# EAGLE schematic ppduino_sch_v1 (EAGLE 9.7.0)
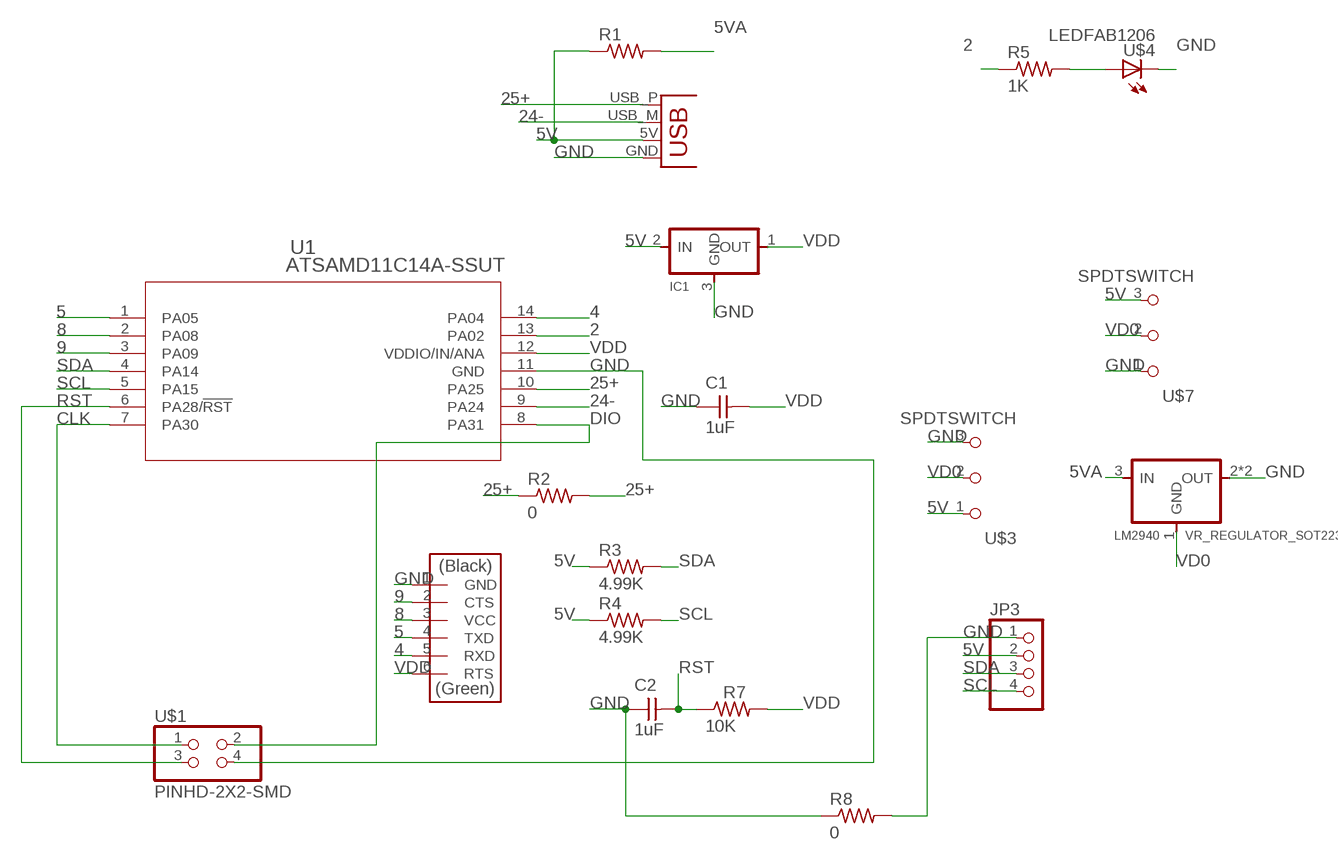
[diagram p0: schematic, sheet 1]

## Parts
C1  1uF  CAP_UNPOLARIZEDFAB  [C1206FAB]
C2  1uF  CAP_UNPOLARIZEDFAB  [C1206FAB]
IC1  VR_REGULATOR-SOT23SOT23  [SOT23]
JP3  PINHD-1X04_2.54-SMD-90°  [1X04SMD/90]
LM2940  VR_REGULATOR_SOT223  [SOT223]
R1  RES-US1206FAB  [R1206FAB]
R2  0  R1206FAB  [R1206FAB]
R3  4.99K  R1206FAB  [R1206FAB]
R4  4.99K  R1206FAB  [R1206FAB]
R5  1K  R1206FAB  [R1206FAB]
R7  10K  R1206FAB  [R1206FAB]
R8  0  R1206FAB  [R1206FAB]
U1  ATSAMD11C14A-SSUT  [SOIC14_SL_MCH]
U$1  PINHD-2X2-SMD  [2X02SMD]
U$3  SPDTSWITCH  [SPDTSWITCH]
U$4  LEDFAB1206  [LED1206FAB]
U$6  CONN_06_FTDI-SMD-HEADER  [1X06SMD]
U$7  SPDTSWITCH  [SPDTSWITCH]
X1  CONN_USBPCB  [USB-A-PCB]

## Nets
2: R5.1 U1.13(PA02)
4: U1.14(PA04) U$6.5(RXD)
5: U1.1(PA05) U$6.4(TXD)
5V: IC1.2(IN) JP3.2 R1.1 R3.1 R4.1 U$3.1 U$7.3 X1.5V(VBUS)
5VA: LM2940.3(IN) R1.2
8: U1.2(PA08) U$6.3(VCC)
9: U1.3(PA09) U$6.2(CTS)
24-: U1.9(PA24) X1.USB_M(D-)
25+: R2.1 R2.2 U1.10(PA25) X1.USB_P(D+)
CLK: U1.7(PA30) U$1.1
DIO: U1.8(PA31) U$1.2
GND: C1.1 C2.1 IC1.3(GND) JP3.1 LM2940.2(OUT) LM2940.4(OUT) R8.1 R8.2 U1.11(GND) U$1.4 U$3.3 U$4.2(C) U$6.1(GND) U$7.1 X1.GND
N$5: R5.2 U$4.1(A)
RST: C2.2 R7.1 U1.6(PA28/!RST) U$1.3
SCL: JP3.4 R4.2 U1.5(PA15)
SDA: JP3.3 R3.2 U1.4(PA14)
VD0: LM2940.1(GND) U$3.2 U$7.2
VDD: C1.2 IC1.1(OUT) R7.2 U1.12(VDDIO/IN/ANA) U$6.6(RTS)

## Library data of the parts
C1 C2 = fab:CAP_UNPOLARIZED
IC1 = fab:VR_REGULATOR-SOT23
JP3 = pinhead-2:PINHD-1X04: PIN HEADER
LM2940 = fab:VR_REGULATOR_SOT223
R1 = fab:RES-US: Resistor (US Symbol)
R2-R5 R7 R8 = fab:R: Resistor (US Symbol)
U1 = samd11c:ATSAMD11C14A-SSUT; BUILT_BY: EMA_Molly; COPYRIGHT: Copyright (C) 2018 Accelerated Designs. All rights reserved; MANUFACTURER_PART_NUMBER: ATSAMD11C14A-SSUT; SOURCELIBRARY: Microchip_2019-08-23_25; VENDOR: Microchip
U$1 = fab:PINHD-2X2-SMD
U$3 U$7 = fab:SPDTSWITCH
U$4 = fab:LED: LED
U$6 = fab:CONN_06_FTDI-SMD-HEADER
X1 = fab:CONN_USB: USB Connectors USB-B-PTH is fully proven SKU : PRT-00139 USB-miniB is fully proven SKU : PRT-00587 USB-A-PCB is untested. USB-A-H is throughly reviewed, but untested. Spark Fun Electronics SKU : PRT-00437 USB-B-SMT is throughly reviewed, but untested. Needs silkscreen touching up. USB-A-S has not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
